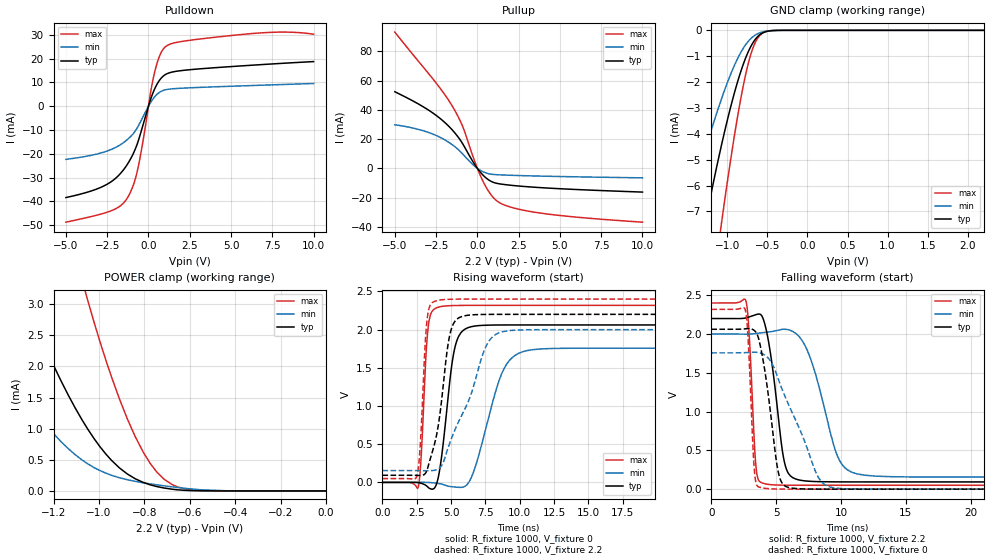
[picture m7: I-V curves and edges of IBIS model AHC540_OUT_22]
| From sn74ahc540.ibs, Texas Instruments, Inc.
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[Model]   AHC540_OUT_22
Model_type  3-state
Enable   Active-Low
Vref =   0
Rref =   1000
Cref =   50p
Vmeas =   1.1
| variable   typ   min   max
C_comp   2.64pF   2.40pF   2.76pF
| C_pullup   3.55pF   2.59pF   4.25pF
| C_pulldown   3.54pF   2.76pF   4.48pF
| C_tri-state   2.64pF   2.40pF   2.76pF
[Temperature Range]   40   100   -40
| Ambient temperature   25   85   -40
[Voltage range]   2.2   2   2.4
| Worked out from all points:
|   slope of the pulldown table from 0 to 0.33 V, typ, clamps not added: 50.4 ohm
|   slope of the pullup table from 0 to 0.33 V, typ, clamps not added: 73 ohm
|   GND clamp passes 1 mA (typ) near -0.76 V on its own axis
|   POWER clamp passes 1 mA (typ) near -1.05 V on its own axis
|   rising waveform, R_fixture 1000, V_fixture 0: 20-80 % time 788ps typ, 1.64ns min, 382ps max; typ from 0 V to 2.06 V
|   falling waveform, R_fixture 1000, V_fixture 2.2: 20-80 % time 927ps typ, 1.76ns min, 403ps max; typ from 2.2 V to 0.093 V
|   rising waveform, R_fixture 1000, V_fixture 2.2: 20-80 % time 947ps typ, 2.3ns min, 389ps max; typ from 0.093 V to 2.2 V
|   falling waveform, R_fixture 1000, V_fixture 0: 20-80 % time 969ps typ, 2.56ns min, 373ps max; typ from 2.06 V to 0 V
[GND Clamp]
| AHC540_OUT_22
|   Voltage   I(typ)   I(min)   I(max)
-5V       -95.67mA   -62.49mA   -121.3mA
-1.555V   -12.25mA   -7.735mA   -19.36mA
-1.505V   -11.34mA   -7.146mA   -18.05mA
-1.28V    -7.515mA   -4.659mA   -12.33mA
-1.075V   -4.462mA   -2.668mA   -7.496mA
-910mV    -2.397mA   -1.344mA   -4.04mA
-775mV    -1.095mA   -569.8uA   -1.756mA
-680mV    -478.4uA   -246.1uA   -680.2uA
-625mV    -252.5uA   -136.6uA   -320.5uA
-565mV    -107.1uA   -65.05uA   -116.6uA
-385mV    -4.065uA   -3.051uA   -2.223uA
2.2V      2.923nA    2.223nA    5.22nA
[POWER Clamp]
| AHC540_OUT_22
|   Voltage   I(typ)   I(min)   I(max)
-5V       75.68mA    48.36mA    122.9mA
-1.595V   5.897mA    3.159mA    12.53mA
-1.345V   3.264mA    1.609mA    7.645mA
-1.315V   2.988mA    1.452mA    7.116mA
-1.195V   1.98mA     900.5uA    5.135mA
-1.075V   1.146mA    499uA      3.398mA
-1.05V    997.5uA    437uA      3.07mA
-945mV    493.1uA    251.9uA    1.835mA
-840mV    195.1uA    153.7uA    871.9uA
-715mV    48.19uA    82.85uA    194.3uA
-590mV    4.147uA    30.5uA     16.16uA
-84.45fV  2.923nA    1.022nA    8.325nA
[Pulldown]
| AHC540_OUT_22
|   Voltage   I(typ)   I(min)   I(max)
-5V       -38.39mA   -22.35mA   -48.74mA
-2.53V    -32.9mA    -18.91mA   -44.61mA
-1.72V    -28.46mA   -16.29mA   -41.96mA
-1.225V   -23.84mA   -13.71mA   -37.94mA
-890mV    -19.48mA   -11.25mA   -32.6mA
-635mV    -14.96mA   -8.551mA   -26.03mA
155mV     3.386mA    1.843mA    6.786mA
405mV     7.696mA    4.159mA    15.11mA
720mV     11.34mA    6.021mA    21.83mA
1.055V    13.39mA    6.916mA    25.12mA
6.265V    17.2mA     8.661mA    30.49mA
10V       18.72mA    9.517mA    30.23mA
[Pullup]
| AHC540_OUT_22
|   Voltage   I(typ)   I(min)   I(max)
-5V       52.39mA    29.77mA    93.2mA
-2.88V    39.25mA    24.22mA    63.76mA
-2.145V   33.06mA    20.54mA    53.11mA
-1.53V    26.37mA    16.21mA    42.8mA
-875mV    16.51mA    9.595mA    28.19mA
-145mV    2.393mA    1.295mA    4.318mA
295mV     -4.104mA   -2.07mA    -7.768mA
745mV     -8.356mA   -3.856mA   -16.81mA
1.2V      -10.33mA   -4.376mA   -22.45mA
2.105V    -11.69mA   -4.798mA   -26.84mA
3.745V    -13.16mA   -5.315mA   -30.51mA
10V       -16.26mA   -6.528mA   -36.86mA
[Ramp]
| AHC540_OUT_22
| variable   typ   min   max
dV/dt_r   1.29/8.23E-10   1.09/1.69E-09   1.44/3.98E-10
dV/dt_f   1.30/9.62E-10   1.14/1.84E-09   1.44/4.17E-10
R_load = 1000
[Rising Waveform]
| AHC540_OUT_22
R_fixture =   1000
C_fixture =   0
L_fixture =   0
V_fixture =   0
V_fixture_min = 0
V_fixture_max = 0
|   Time   V(typ)   V(min)   V(max)
0s        1.402nV    2.451nV    738pV
2.6ns     -2.859mV   728.9uV    -66.53mV
2.805ns   -10.8mV    721.9uV    292.5mV
3.325ns   -63.64mV   -571.8uV   2.02V
4.135ns   127.6mV    -15.85mV   2.297V
5.245ns   1.739V     -59.97mV   2.316V
6.475ns   2.038V     64.7mV     2.317V
8.72ns    2.061V     1.436V     2.317V
10.52ns   2.061V     1.725V     2.317V
50ns      2.061V     1.757V     2.317V
[Falling Waveform]
| AHC540_OUT_22
R_fixture =   1000
C_fixture =   0
L_fixture =   0
V_fixture =   2.2
V_fixture_min = 2
V_fixture_max = 2.4
|   Time   V(typ)   V(min)   V(max)
0s        2.2V       2V         2.4V
2.665ns   2.208V     1.999V     2.426V
2.905ns   2.22V      1.999V     2.031V
3.45ns    2.251V     2.007V     279mV
4.07ns    2.16V      2.019V     72.64mV
5.615ns   363.4mV    2.062V     51.52mV
6.66ns    122.9mV    1.987V     50.45mV
9.735ns   94.04mV    423.4mV    50.2mV
11.21ns   93.44mV    198.3mV    50.2mV
50ns      93.27mV    155.2mV    50.2mV
[Rising Waveform]
| AHC540_OUT_22
R_fixture =   1000
C_fixture =   0
L_fixture =   0
V_fixture =   2.2
V_fixture_min = 2
V_fixture_max = 2.4
|   Time   V(typ)   V(min)   V(max)
0s        93.27mV    155.2mV    50.2mV
2.5ns     91.94mV    155mV      77.51mV
2.745ns   89.96mV    154.5mV    458.6mV
3.26ns    167.9mV    153.1mV    2.142V
3.975ns   649.2mV    168.7mV    2.379V
4.765ns   1.79V      443.8mV    2.396V
5.2ns     2.087V     654.1mV    2.398V
7.565ns   2.199V     1.789V     2.4V
8.815ns   2.2V       1.975V     2.4V
50ns      2.2V       2V         2.4V
[Falling Waveform]
| AHC540_OUT_22
R_fixture =   1000
C_fixture =   0
L_fixture =   0
V_fixture =   0
V_fixture_min = 0
V_fixture_max = 0
|   Time   V(typ)   V(min)   V(max)
0s        2.061V     1.757V     2.317V
2.63ns    2.067V     1.76V      2.304V
2.83ns    2.071V     1.762V     1.95V
3.31ns    2.046V     1.765V     261.8mV
3.71ns    1.899V     1.758V     25.08mV
5.145ns   233.9mV    1.427V     1.712mV
5.985ns   20.72mV    1.078V     438.7uV
8.225ns   768.8uV    160.2mV    15.41uV
9.485ns   171.4uV    15.95mV    2.621uV
50ns      -2.901nV   5.94nV     9.71nV
